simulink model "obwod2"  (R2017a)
settings: Solver=VariableStepAuto  StartTime=0.0  StopTime=100.0  RelTol=1e-6
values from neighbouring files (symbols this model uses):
  dx1 = w1/(1-K1*K2)    (= 0.616649537513)    [obwod2m.m]    (also in cz1.m; cz1m.m; obwod1m.m; obwod3m.m = 0.6)
  dx2 = 1/(T1*(1-K1*K2))    (= 0.0513874614594)    [obwod2m.m]    (also in cz1.m = 1.02774922919; cz1m.m = 1.02774922919; obwod1m.m = 1.02774922919; obwod3m.m = 0.05)
  dx3 = (w2*K1)/(1-K1*K2)    (= 0.172045220966)    [obwod2m.m]    (also in cz1.m; cz1m.m; obwod1m.m; obwod3m.m = 0)
  dx4 = K1/(T2*(1-K1*K2))    (= 0.013874614594)    [obwod2m.m]    (also in cz1.m = 0.277492291881; cz1m.m = 0.277492291881; obwod1m.m = 0.277492291881; obwod3m.m = 0)
  dx5 = 1/(L1*(1-K1*K2))    (= 1.02774922919)    [obwod2m.m]    (also in cz1.m; cz1m.m; obwod1m.m; obwod3m.m = 1)
  ex1 = (w2*K2)/(1-K1*K2)    (= 0.0637204522097)    [obwod2m.m]    (also in cz1.m; cz1m.m; obwod1m.m; obwod3m.m = 0)
  ex2 = K2/(T1*(1-K1*K2))    (= 0.00513874614594)    [obwod2m.m]    (also in cz1.m = 0.102774922919; cz1m.m = 0.102774922919; obwod1m.m = 0.102774922919; obwod3m.m = 0)
  ex3 = w2/(1-K1*K2)    (= 0.637204522097)    [obwod2m.m]    (also in cz1.m; cz1m.m; obwod1m.m; obwod3m.m = 0.62)
  ex4 = 1/(T2*(1-K1*K2))    (= 0.0513874614594)    [obwod2m.m]    (also in cz1.m = 1.02774922919; cz1m.m = 1.02774922919; obwod1m.m = 1.02774922919; obwod3m.m = 0.05)
  ex5 = (K2*1)/(L1*(1-K1*K2))    (= 0.102774922919)    [obwod2m.m]    (also in cz1.m; cz1m.m; obwod1m.m; obwod3m.m = 0)

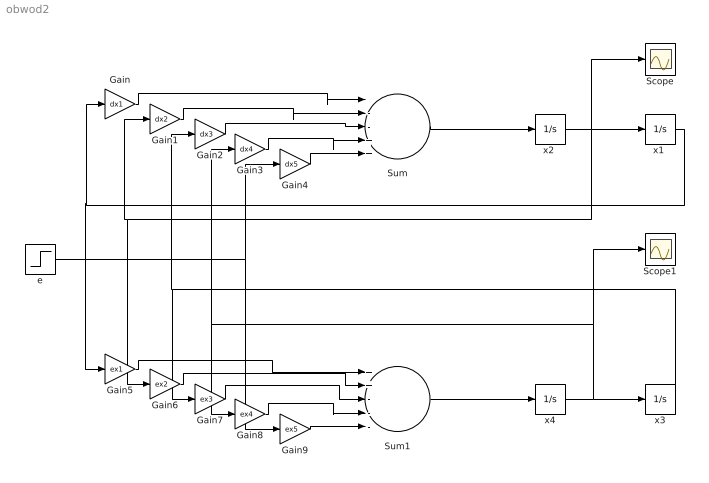
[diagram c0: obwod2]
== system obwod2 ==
  Gain : Gain  Gain=dx1
  Gain1 : Gain  Gain=dx2
  Gain2 : Gain  Gain=dx3
  Gain3 : Gain  Gain=dx4
  Gain4 : Gain  Gain=dx5
  Gain5 : Gain  Gain=ex1
  Gain6 : Gain  Gain=ex2
  Gain7 : Gain  Gain=ex3
  Gain8 : Gain  Gain=ex4
  Gain9 : Gain  Gain=ex5
  Scope : Scope
  Scope1 : Scope
  Sum : Sum  Inputs=|--+++
  Sum1 : Sum  Inputs=++---
  e : Step  Time=0  After=10  SampleTime=0
  "x1 " : Integrator
  "x2 " : Integrator
  x3 : Integrator
  x4 : Integrator
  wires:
  Sum/1 -> "x2 "/1
  "x2 "/1 -> Scope/1, Gain6/1, Gain1/1, "x1 "/1
  Gain4/1 -> Sum/5
  Gain3/1 -> Sum/4
  Gain2/1 -> Sum/3
  Gain1/1 -> Sum/2
  Gain/1 -> Sum/1
  "x1 "/1 -> Gain5/1, Gain/1
  Sum1/1 -> x4/1
  x4/1 -> Gain8/1, Gain3/1, Scope1/1, x3/1
  e/1 -> Gain4/1, Gain9/1
  Gain9/1 -> Sum1/5
  Gain8/1 -> Sum1/4
  Gain7/1 -> Sum1/3
  Gain6/1 -> Sum1/2
  Gain5/1 -> Sum1/1
  x3/1 -> Gain7/1, Gain2/1
